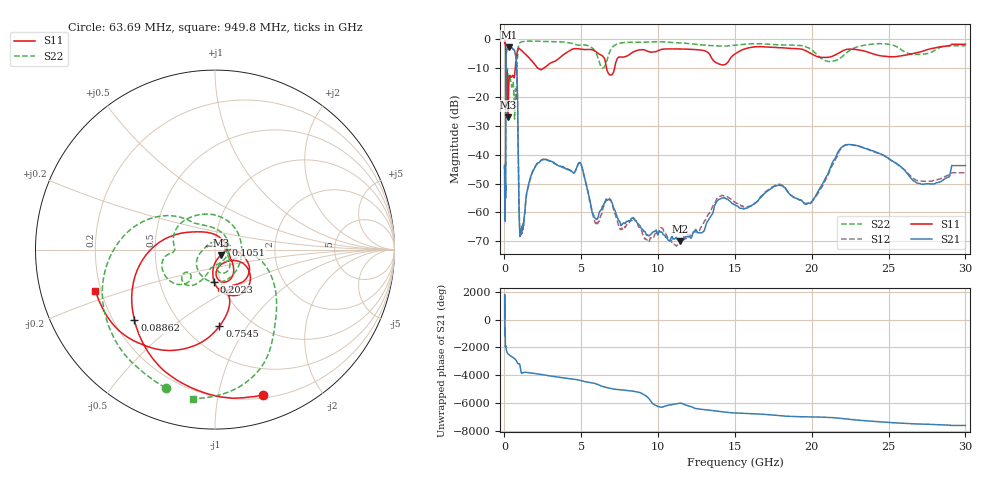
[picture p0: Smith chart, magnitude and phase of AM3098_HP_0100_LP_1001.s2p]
! Date/Time: Thu, Feb 28, 2019 8:35 AM
! Network Analyzer: Agilent Technologies E8364B Rev: A.07.50.67
! Sweep from 0.010 to 30.000 GHz, 1601 Points, Sweep Type: LOG
! Power Supply: 5.022 V, 0.002 A
# Hz S DB R 50
!freq MagS11 AngS11 MagS21 AngS21 MagS12 AngS12 MagS22 AngS22
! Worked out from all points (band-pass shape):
!   1601 points, 10 MHz to 30 GHz, reference 50 ohm
!   highest |S21| = -2.78 dB at 299 MHz (marker M1); lowest = -70.0 dB at 11.42 GHz (marker M2)
!   |S21| within 3 dB of the highest: 112.1 MHz to 735.4 MHz (623.3 MHz wide, 147 % of centre)
!   lowest |S11| = -27.0 dB at 236.3 MHz (marker M3), VSWR 1.09, Z = 53.3 - j3.24 ohm
!   |S11| at or under -10 dB: 95.97 MHz to 701.8 MHz (605.9 MHz wide, 152 % of centre); 2.191 GHz to 2.548 GHz (357.1 MHz wide, 15.1 % of centre); 6.646 GHz to 7.167 GHz (521.2 MHz wide, 7.55 % of centre)
!   |S22| runs from -27.6 to -0.5 dB; largest |S21 - S12| = 0.013
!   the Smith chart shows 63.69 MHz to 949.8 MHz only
!   S11 on the Smith chart (normalised r, x): 63.69 MHz: 0.23, -1.35; 88.62 MHz: 0.29, -0.35; 105.1 MHz: 1.13, +0.06; 202.3 MHz: 0.93, -0.34; 754.5 MHz: 0.72, -0.75; 949.8 MHz: 0.18, -0.16
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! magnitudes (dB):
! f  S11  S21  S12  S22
! 10 MHz  -0.3  -44.7  -43.1  -0.6
! 38.04 MHz  -0.5  -58.4  -59.1  -1.0
! 63.69 MHz  -1.4  -52.0  -51.9  -1.8
! 77.03 MHz  -2.2  -49.1  -53.1  -2.6
! 88.62 MHz  -4.5  -32.6  -32.1  -4.9
! 105.1 MHz  -23.7  -7.7  -7.7  -19.6
! 144.7 MHz  -16.9  -3.6  -3.5  -13.6
! 202.3 MHz  -15.0  -3.1  -3.1  -10.9
! 236.3 MHz  -27.0  -2.9  -2.8  -12.6
! 299 MHz  -14.1  -2.8  -2.7  -12.5
! 550.5 MHz  -12.5  -3.3  -3.3  -14.8
! 754.5 MHz  -7.4  -6.6  -6.6  -21.3
! 838.1 MHz  -4.1  -17.0  -17.0  -7.2
! 949.8 MHz  -3.0  -58.7  -58.5  -1.5
! 1.149 GHz  -4.0  -66.0  -64.9  -0.8
! 2.084 GHz  -9.4  -43.4  -43.4  -0.6
! 4.903 GHz  -3.3  -42.7  -42.8  -2.0
! 7.926 GHz  -5.9  -63.1  -64.6  -1.0
! 11.42 GHz  -3.3  -70.0  -70.5  -1.2
! 19.7 GHz  -4.2  -57.1  -56.8  -2.7
! 22.67 GHz  -3.4  -36.6  -36.7  -3.2
! 30 GHz  -1.7  -43.8  -46.2  -2.2
